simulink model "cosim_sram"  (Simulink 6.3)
settings: Solver=ode45  StartTime=0.0  StopTime=200.0  RelTol=1e-3
undefined symbols (not defined in the file or in its folder): netlist, test_sram_top
libraries: sram_cosim_lib x1, simulink x1

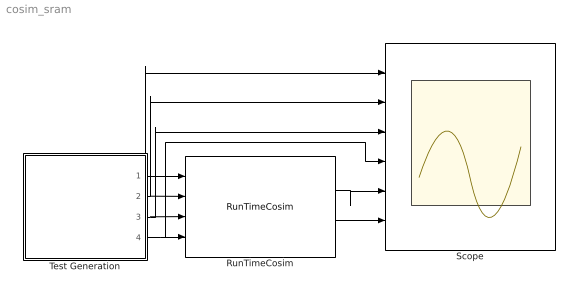
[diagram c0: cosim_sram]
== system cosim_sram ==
  RunTimeCosim : sram_cosim_lib/RunTimeCosim  index=0  bitstream=netlist/test_sram_top.bit  freq=90  single_step=on  shared=None
  Scope : Scope  NumInputPorts=6
  Test Generation : Subsystem
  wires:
  Test Generation/1(d) -> RunTimeCosim/1, Scope/1
  Test Generation/2(a) -> RunTimeCosim/2, Scope/2
  Test Generation/3(w) -> RunTimeCosim/3, Scope/3
  Test Generation/4(r) -> RunTimeCosim/4, Scope/4
  RunTimeCosim/1 -> Scope/5
  RunTimeCosim/2 -> Scope/6

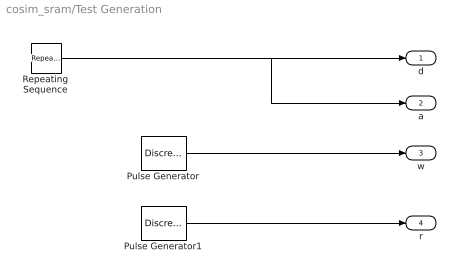
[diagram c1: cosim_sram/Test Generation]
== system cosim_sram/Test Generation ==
  Pulse Generator : DiscretePulseGenerator  PulseType=Time based  Period=128  PulseWidth=25
  Pulse Generator1 : DiscretePulseGenerator  PulseType=Time based  Period=128  PulseWidth=25  PhaseDelay=63
  Repeating Sequence : simulink/Sources/Repeating Sequence  rep_seq_t=[1:64]  rep_seq_y=[0:63]
  d : Outport
  a : Outport  Port=2
  w : Outport  Port=3
  r : Outport  Port=4
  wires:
  Pulse Generator1/1 -> r/1
  Pulse Generator/1 -> w/1
  Repeating Sequence/1 -> a/1, d/1
